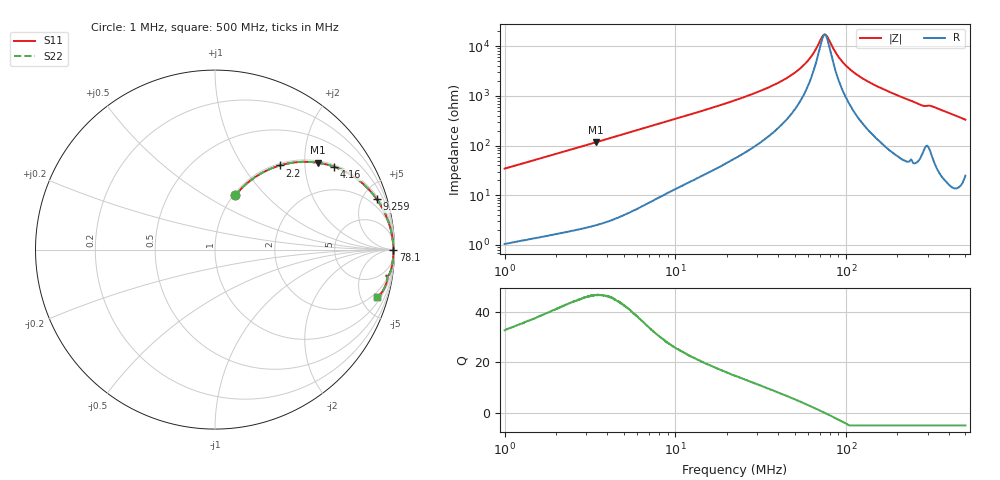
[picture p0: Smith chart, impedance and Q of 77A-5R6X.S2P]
!s-Parameter Generated by FASTRON Sdn. Bhd.
!FASTRON P/N : 77A-5R6X
!Keysight Technologies,E4991B,MY54100416,A.01.15
!Date: Mon Mar 16 11:26:04 2026
!Version  : Rev00 Mon Mar 16 11:26:04 2026
!Data & Calibration Information:
!PortZ  Port1:50+j0  Port2:50+j0
!When reading, reference impedance value at option line is always used.
! Remarks : This data is being provided solely for informational purposes.
!Freq	S11	S21	S12	S22
# Hz S dB R 50
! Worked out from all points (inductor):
!   1601 points, 1 MHz to 500 MHz, reference 50 ohm
!   read as one part in series: L = 5.44 uH near 1.032 MHz
!   highest Q = 46.7 at 3.439 MHz (marker M1), where L = 5.4 uH
!   self-resonance near 74.83 MHz
!   S11 on the Smith chart (normalised r, x): 1 MHz: 1.02, +0.69; 2.2 MHz: 1.04, +1.50; 4.16 MHz: 1.06, +2.83; 9.259 MHz: 1.23, +6.34; 78.1 MHz: open; 500 MHz: 1.50, -6.62
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1000000  -9.84 69.5  -0.57 -18.8  -0.57 -18.8  -9.84 69.5
2200046  -4.55 52.3  -2.03 -36.3  -2.03 -36.3  -4.55 52.3
2820919  -3.30 45.6  -2.92 -43.2  -2.92 -43.2  -3.30 45.6
3438906  -2.48 40.1  -3.83 -48.7  -3.83 -48.7  -2.48 40.1
4159836  -1.85 34.9  -4.86 -53.9  -4.86 -53.9  -1.85 34.9
7957584  -0.64 19.9  -9.34 -68.2  -9.34 -68.2  -0.64 19.9
9259097  -0.50 17.3  -10.53 -70.6  -10.53 -70.6  -0.50 17.3
2.236068e7  -0.14 6.9  -18.36 -79.2  -18.36 -79.2  -0.14 6.9
3.310225e7  -0.09 4.2  -22.71 -80.3  -22.71 -80.3  -0.09 4.2
4.412501e7  -0.07 2.6  -26.90 -79.2  -26.90 -79.2  -0.07 2.6
5.42111e7  -0.06 1.5  -31.24 -75.6  -31.24 -75.6  -0.06 1.5
6.307767e7  -0.05 0.8  -36.30 -66.2  -36.30 -66.2  -0.05 0.8
7.310989e7  -0.05 0.1  -44.20 -19.6  -44.20 -19.6  -0.05 0.1
7.541731e7  -0.05 -0.0  -44.67 4.3  -44.67 4.3  -0.05 -0.0
7.81003e7  -0.05 -0.2  -43.56 29.7  -43.56 29.7  -0.05 -0.2
9.01709e7  -0.05 -0.9  -35.83 68.9  -35.83 68.9  -0.05 -0.9
1.045122e8  -0.05 -1.6  -30.96 77.1  -30.96 77.1  -0.05 -1.6
1.299065e8  -0.06 -2.7  -26.39 80.7  -26.39 80.7  -0.06 -2.7
1.77937e8  -0.08 -4.7  -21.78 81.5  -21.78 81.5  -0.08 -4.7
2.72785e8  -0.21 -8.5  -16.62 76.6  -16.62 76.6  -0.21 -8.5
3.161702e8  -0.25 -8.9  -16.13 75.0  -16.13 75.0  -0.25 -8.9
5e8  -0.55 -16.4  -10.98 69.3  -10.98 69.3  -0.55 -16.4
